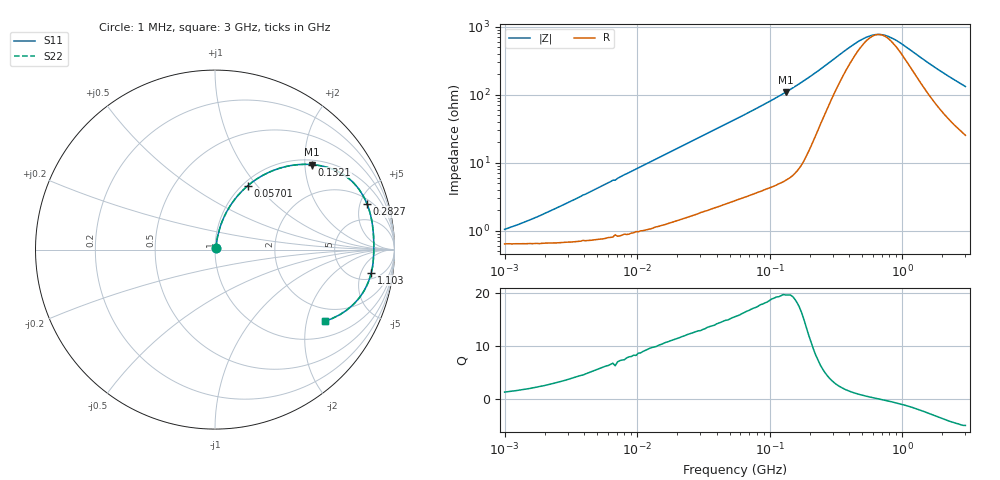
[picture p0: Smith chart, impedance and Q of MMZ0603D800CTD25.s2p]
! S-parameter Generated by TDK Corporation
! Copyright(C) 2018 TDK Corporation.
! All Rights Reserved.
! TDK P/N: MMZ0603D800CTD25 (Chip Bead)
! Property: |Z|=80¶ at 100MHz
! Size(LxWxT): 0.6x0.3x0.3mm, 0.024x0.012x0.012inches
! Model Type: s2p (Touchstone File Format Version 1.0)
! Frequency: DC=Yes Start=1MHz Stop=3000MHz 202points Log-sweep
! Model Generated on Aug. 6, 2018
! Port Assignments:
!  1 ---@@@--- 2
! Applicable Conditions:
!  Temperature = 25 degC
!  DC Bias Current = 0 A
!  Small Signal Operation
! Terms and conditions regarding TDK Simulation Models
! (1)This simulation model is being provided solely for informational purposes. Please refer to the specifications of the products in terms of detailed characteristics of such products.
! (2)In no event shall TDK Corporation of any of its subsidiaries be liable for any loss or damage arising, directly or indirectly,
!  From any information contained in this simulation model, including, but not limited to loss or damages arising from any inaccuracies, omissions or errors in connection with such information.
! (3)Any and all copyrights on this simulation model are owned by TDK Corporation.
!  Duplication or redistribution of this simulation model without prior written permission from TDK Corporation is prohibited.
! (4)This simulation model is subject to any modification or change without any prior notice.
! (5)Neither TDK Corporation nor any of its subsidiaries shall make any warranty, express or implied,
!  Including but not limited to the correctness, implied warranties of merchantability and fitness for a particular purpose with respect to this simulation models.
! (6)The use of this simulation model shall be deemed to have consented to the terms and conditions hereof.
# Hz S MA R 50
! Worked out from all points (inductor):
!   201 points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, 1 MHz to 3 GHz, reference 50 ohm
!   read as one part in series: L = 133 nH near 2.413 MHz
!   highest Q = 19.6 at 132.1 MHz (marker M1), where L = 131 nH
!   self-resonance near 666 MHz
!   S11 on the Smith chart (normalised r, x): 1 MHz: 1.01, +0.02; 57.01 MHz: 1.06, +0.90; 132.1 MHz: 1.11, +2.17; 282.7 MHz: 2.48, +5.78; 1.103 GHz: 7, -8; 3 GHz: 1.51, -2.59
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1000000  0.01046 51.9  0.9936 -0.5  0.9936 -0.5  0.01046 51.9
1822989  0.01642 66.0  0.9934 -0.9  0.9934 -0.9  0.01642 66.0
3900413  0.03327 75.6  0.9923 -1.9  0.9923 -1.9  0.03327 75.6
6563319  0.05491 78.5  0.9905 -3.1  0.9905 -3.1  0.05491 78.5
6831390  0.05493 77.8  0.9899 -3.1  0.9899 -3.1  0.05493 77.8
1.461624e7  0.1171 77.7  0.9817 -6.7  0.9817 -6.7  0.1171 77.7
3.127247e7  0.2377 71.9  0.9534 -13.7  0.9534 -13.7  0.2377 71.9
5.477226e7  0.3877 63.6  0.8972 -22.8  0.8972 -22.8  0.3877 63.6
5.700937e7  0.4007 62.8  0.8911 -23.6  0.8911 -23.6  0.4007 62.8
8.507507e7  0.5452 53.8  0.8083 -33.0  0.8083 -33.0  0.5452 53.8
1.321429e8  0.7182 41.3  0.6602 -45.8  0.6602 -45.8  0.7182 41.3
1.680187e8  0.8029 33.4  0.5516 -53.3  0.5516 -53.3  0.8029 33.4
2.136344e8  0.8589 25.3  0.4299 -58.7  0.4299 -58.7  0.8589 25.3
2.827291e8  0.8845 16.7  0.2965 -59.0  0.2965 -59.0  0.8845 16.7
4.219165e8  0.8874 7.5  0.1668 -43.9  0.1668 -43.9  0.8874 7.5
5.364635e8  0.8859 3.4  0.1267 -24.1  0.1267 -24.1  0.8859 3.4
6.553423e8  0.8848 0.2  0.1153 -1.9  0.1153 -1.9  0.8848 0.2
8.005644e8  0.8842 -2.9  0.125 20.6  0.125 20.6  0.8842 -2.9
1.10276e9  0.8803 -8.4  0.1821 44.8  0.1821 44.8  0.8803 -8.4
1.782824e9  0.8452 -18.9  0.3394 53.8  0.3394 53.8  0.8452 -18.9
2.266846e9  0.8039 -25.1  0.4367 51.4  0.4367 51.4  0.8039 -25.1
3e9  0.7321 -33.0  0.5549 45.9  0.5549 45.9  0.7321 -33.0
